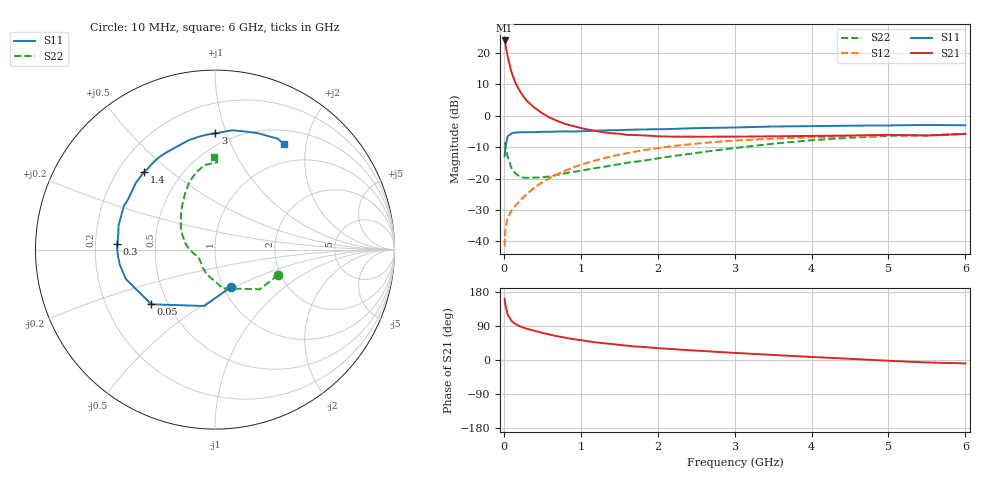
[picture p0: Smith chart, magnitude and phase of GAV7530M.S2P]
! Infineon Technologies  Discrete & RF Semiconductors
! BF775
! Si NPN RF Bipolar Junction Transistor in SOT23
! VCE = 0.75 V  IC = 30 mA
! Common Emitter S-Parameters:  May  1996
# GHz  S  MA  R  50
!  f  S11  S21  S12  S22
! GHz  MAG  ANG  MAG  ANG  MAG  ANG  MAG  ANG
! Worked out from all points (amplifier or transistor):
!   36 points, 10 MHz to 6 GHz, reference 50 ohm
!   highest |S21| = 23.9 dB at 10 MHz (marker M1)
!   |S21| within 3 dB of that: start of sweep to 33.79 MHz
!   unconditionally stable (mu >= 1): start of sweep to end of sweep
!   at 250 MHz: K = 3.48, MAG = 7.8 dB, |S12| = -26.1 dB
!   at 1.4 GHz: K = 2.86, MAG = -3.8 dB, |S12| = -13.0 dB
!   at 6 GHz: K = 1.19, MAG = -2.6 dB, |S12| = -5.8 dB
!   S11 on the Smith chart (normalised r, x): 10 MHz: 1.09, -0.48; 50 MHz: 0.40, -0.32; 300 MHz: 0.29, +0.03; 1.4 GHz: 0.31, +0.41; 3 GHz: 0.41, +0.91; 6 GHz: 0.70, +1.62
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0.01  0.2261 -66.9  15.67 161.7  0.0084 64.5  0.3783 -22.1
0.02  0.3199 -100.8  13.69 146.1  0.0152 58.2  0.3333 -41.6
0.05  0.4682 -139.4  8.662 119.9  0.0241 45.0  0.2202 -78.4
0.1  0.5231 -161.7  4.872 103.2  0.0308 46.0  0.1455 -108.1
0.15  0.5369 -170.9  3.323 94.9  0.0368 50.1  0.1204 -125.4
0.2  0.542 -176.3  2.556 89.8  0.043 54.7  0.109 -134.8
0.25  0.545 179.5  2.052 85.8  0.0497 57.7  0.1037 -141.9
0.3  0.5455 176.6  1.711 82.5  0.0568 60.7  0.1024 -147.1
0.4  0.5461 170.3  1.331 76.9  0.0719 63.2  0.1036 -154.5
0.5  0.5533 166.5  1.09 71.8  0.0869 64.7  0.1043 -159.4
0.6  0.5547 162.1  0.924 66.8  0.1027 64.8  0.1081 -162.8
0.8  0.5625 154.6  0.737 58.9  0.1336 63.7  0.1214 -170.0
1.1  0.5696 142.8  0.599 49.3  0.18 60.4  0.1403 -179.2
1.4  0.5867 132.4  0.524 42.2  0.2246 55.7  0.1613 171.0
1.7  0.5997 122.7  0.492 35.7  0.2658 50.6  0.1848 160.7
2.2  0.6143 108.9  0.463 28.7  0.3277 41.7  0.2279 146.6
2.6  0.6352 98.3  0.462 23.7  0.3679 34.6  0.2649 135.8
3  0.6475 89.9  0.463 18.8  0.4012 27.8  0.3054 126.8
3.5  0.6717 81.8  0.469 13.3  0.431 19.9  0.3574 117.7
4.5  0.6919 69.4  0.483 3.1  0.4708 6.8  0.4443 103.3
5.5  0.7105 60.6  0.483 -6.5  0.4822 -4.7  0.4866 88.5
6  0.7015 56.9  0.512 -9.0  0.5109 -8.2  0.5142 90.8
